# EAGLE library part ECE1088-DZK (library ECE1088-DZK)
Interface - I/O Expanders GPIO EXPANSION SMbus Source: Datasheet
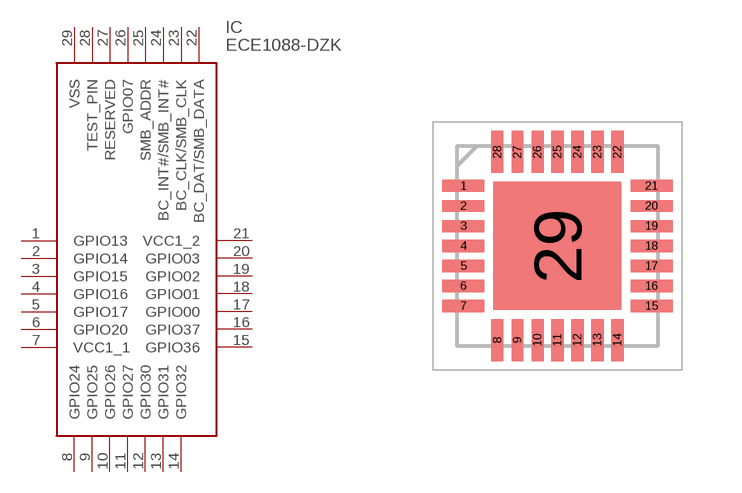
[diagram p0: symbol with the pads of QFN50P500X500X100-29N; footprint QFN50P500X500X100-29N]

Designator prefix IC

## ECE1088-DZK (Arrow_Part_Number: ECE1088-DZK; Arrow_Price-Stock: https://www.arrow.com/en/products/ece1088-dzk/microchip-technology?region=nac; Description: Interface - I/O Expanders GPIO EXPANSION SMbus; Height: 1mm; Manufacturer_Name: Microchip; Manufacturer_Part_Number: ECE1088-DZK; Mouser_Part_Number: 886-ECE1088-DZK; Mouser_Price-Stock: https://www.mouser.co.uk/ProductDetail/Microchip-Technology/ECE1088-DZK?qs=pA5MXup5wxED3mV%2FEJAOBQ%3D%3D)  [QFN50P500X500X100-29N]
1  GPIO13
2  GPIO14
3  GPIO15
4  GPIO16
5  GPIO17
6  GPIO20
7  VCC1_1
8  GPIO24
9  GPIO25
10  GPIO26
11  GPIO27
12  GPIO30
13  GPIO31
14  GPIO32
15  GPIO36
16  GPIO37
17  GPIO00
18  GPIO01
19  GPIO02
20  GPIO03
21  VCC1_2
22  BC_DAT/SMB_DATA
23  BC_CLK/SMB_CLK
24  BC_INT#/SMB_INT#
25  SMB_ADDR
26  GPIO07
27  RESERVED
28  TEST_PIN
29  VSS

## Footprint QFN50P500X500X100-29N (pad centres in mm)
28 TERMINAL QFN 5X5MM BODY 0.5MM PITCH
smd 1.05 x 0.3: 1 -2.35,1.5; 2 -2.35,1; 3 -2.35,0.5; 4 -2.35,0; 5 -2.35,-0.5; 6 -2.35,-1; 7 -2.35,-1.5; 15 2.35,-1.5; 16 2.35,-1; 17 2.35,-0.5; 18 2.35,0; 19 2.35,0.5; 20 2.35,1; 21 2.35,1.5
smd 0.3 x 1.05: 8 -1.5,-2.35; 9 -1,-2.35; 10 -0.5,-2.35; 11 0,-2.35; 12 0.5,-2.35; 13 1,-2.35; 14 1.5,-2.35; 22 1.5,2.35; 23 1,2.35; 24 0.5,2.35; 25 0,2.35; 26 -0.5,2.35; 27 -1,2.35; 28 -1.5,2.35
smd 3.2 x 3.2: 29 0,0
